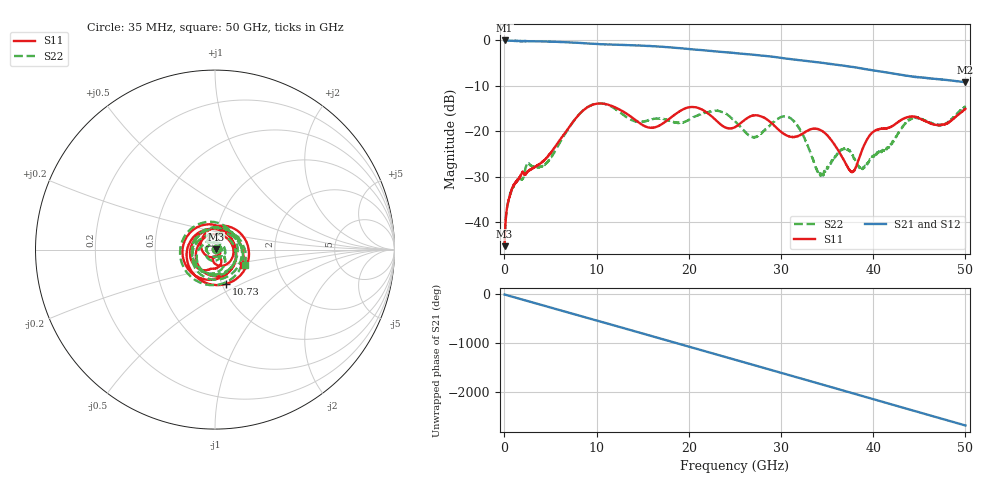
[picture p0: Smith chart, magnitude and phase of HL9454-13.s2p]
! 3/7/2022 11:42:01 AM
! H:\PRODUCTION_DATA\TEMP_S2P.S2P
! CHANNEL.1
! TR.MEASUREMENT
! CORRECTED.DATA
# GHZ S RI R 50.0
! FREQ.GHZ  S11RE  S11IM  S21RE  S21IM  S12RE  S12IM  S22RE  S22IM
!; PortSelection: Port_12
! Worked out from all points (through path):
!   3571 points, 35 MHz to 50 GHz, reference 50 ohm
!   highest |S21| = -0.04 dB at 35 MHz (marker M1); lowest = -9.2 dB at 49.97 GHz (marker M2)
!   group delay of S21, straight-line fit = 149 ps
!   lowest |S11| = -45.3 dB at 35 MHz (marker M3), VSWR 1.01, Z = 50.5 + j0.278 ohm
!   |S11| at or under -10 dB: start of sweep to end of sweep
!   |S22| runs from -45.1 to -13.9 dB; largest |S21 - S12| = 0.0091
!   S11 on the Smith chart (normalised r, x): 35 MHz: 1.01, +0.01; 10.73 GHz: 1.05, -0.42; 50 GHz: 1.34, -0.23
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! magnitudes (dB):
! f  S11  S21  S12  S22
! 35 MHz  -45.3  0.0  0.0  -45.1
! 440.9 MHz  -35.3  -0.1  -0.1  -35.4
! 1.113 GHz  -31.6  -0.1  -0.1  -31.6
! 2.54 GHz  -28.8  -0.2  -0.2  -27.1
! 4.57 GHz  -25.9  -0.3  -0.3  -27.0
! 8.376 GHz  -15.8  -0.6  -0.6  -15.8
! 10.73 GHz  -13.9  -0.9  -0.9  -13.9
! 16.7 GHz  -18.8  -1.4  -1.4  -17.2
! 20.4 GHz  -14.7  -2.0  -2.0  -17.0
! 25.03 GHz  -19.1  -2.8  -2.8  -17.8
! 27.12 GHz  -16.5  -3.2  -3.2  -21.3
! 30.87 GHz  -21.1  -4.1  -4.1  -16.9
! 33.36 GHz  -19.5  -4.7  -4.7  -25.7
! 34.39 GHz  -19.9  -4.9  -5.0  -29.6
! 36.52 GHz  -25.3  -5.5  -5.5  -24.1
! 37.71 GHz  -29.0  -5.9  -5.9  -25.2
! 38.83 GHz  -24.0  -6.2  -6.2  -28.2
! 41.69 GHz  -19.2  -7.1  -7.1  -23.6
! 44.11 GHz  -16.8  -7.9  -7.9  -17.2
! 47.52 GHz  -18.6  -8.7  -8.6  -18.7
! 49.97 GHz  -15.1  -9.2  -9.2  -14.6
! 50 GHz  -15.1  -9.2  -9.2  -14.5
